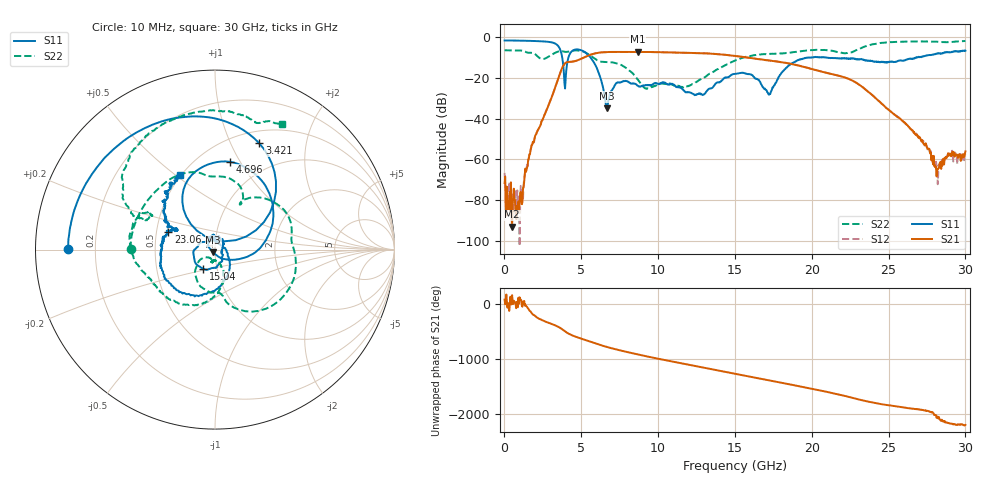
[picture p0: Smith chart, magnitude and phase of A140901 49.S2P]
!  2-Port S-parameters saved by WinCal
! VAR MeasName=S-Parameters (CALIBRATED_DATA) read from VNA (N5244A)
! VAR MeasDate=11/3/2014 9:34:34 AM
! VAR NAME=A140901 49
! VAR FILENAME=A140901 49.S2P
! VAR DATE=11/3/2014 9:34:34 AM
! VAR PHYS_PORTS=1,2
# Hz S RI R 50
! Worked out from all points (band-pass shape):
!   801 points, 10 MHz to 30 GHz, reference 50 ohm
!   highest |S21| = -7.30 dB at 8.67 GHz (marker M1); lowest = -93.0 dB at 497.3 MHz (marker M2)
!   |S21| within 3 dB of the highest: 5.111 GHz to 16 GHz (10.89 GHz wide, 103 % of centre)
!   lowest |S11| = -35.0 dB at 6.645 GHz (marker M3), VSWR 1.04, Z = 49 - j1.43 ohm
!   |S11| at or under -10 dB: 3.757 GHz to 4.167 GHz (410 MHz wide, 10.4 % of centre); 5.593 GHz to 20.06 GHz (14.47 GHz wide, 113 % of centre); 20.8 GHz to 26.84 GHz (6.04 GHz wide, 25.4 % of centre)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
!   |S22| runs from -25.4 to -2.0 dB; largest |S21 - S12| = 0.0038
!   S11 on the Smith chart (normalised r, x): 10 MHz: 0.10, +0.00; 3.421 GHz: 0.64, +1.29; 4.696 GHz: 0.70, +0.90; 15.04 GHz: 0.86, -0.19; 23.06 GHz: 0.58, +0.12; 30 GHz: 0.49, +0.52
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1e7  -0.8177 0.00209  7.3e-06 0.000264  0.00033 0.000331  -0.4708 0.00438
4.973375e8  -0.7992 0.1616  -2.19e-05 4.15e-06  -5.05e-05 0.000124  -0.4113 0.2191
1.05965e9  -0.7361 0.3355  6.56e-06 0.00016  1.52e-05 0.000224  -0.2331 0.402
1.734425e9  -0.6 0.526  -0.00154 -0.00114  -0.00151 -0.00119  0.0341 0.4071
3.421362e9  0.2467 0.5922  0.0621 -0.0466  0.0623 -0.0466  0.3434 0.2548
3.946188e9  -0.0046 0.0543  -0.1504 -0.1685  -0.1507 -0.1682  0.4259 0.0644
4.695938e9  0.0815 0.4893  -0.1515 0.2138  -0.1513 0.2136  0.4282 -0.1876
5.033325e9  0.257 0.3878  -0.0136 0.2958  -0.0139 0.2952  0.3298 -0.3053
5.933025e9  0.1966 -0.031  0.3938 0.0516  0.3934 0.0523  0.0544 -0.2786
6.645288e9  -0.0103 -0.0146  0.253 -0.3406  0.253 -0.3401  0.0115 -0.2409
8.669612e9  -0.000731 0.0642  -0.4232 0.0849  -0.4227 0.0843  -0.0753 -0.0505
1.001916e10  0.00609 0.0707  0.00649 0.4235  0.0065 0.4224  -0.0168 -0.0671
1.155615e10  0.0455 0.0284  0.4084 0.0303  0.4084 0.0308  -0.00548 -0.0591
1.305565e10  0.0363 -0.0202  0.0878 -0.3873  0.0867 -0.3867  0.0362 -0.0971
1.5005e10  -0.0603 -0.1082  -0.3412 0.0266  -0.3407 0.0278  -0.00464 -0.2635
1.504249e10  -0.0647 -0.1073  -0.3388 0.0383  -0.3387 0.0393  -0.0104 -0.265
1.725425e10  0.027 0.0301  0.1485 0.2191  0.1455 0.2185  -0.301 -0.2388
2.002832e10  -0.2529 -0.1863  -0.0279 -0.1599  -0.0272 -0.1609  -0.4734 0.0296
2.306481e10  -0.2601 0.0985  0.0264 0.0628  0.0261 0.0634  -0.4611 0.1994
2.501416e10  -0.211 0.1129  0.0128 -0.0101  0.0129 -0.0102  -0.3863 0.6314
2.812562e10  -0.2842 0.2622  -1.8e-05 0.00038  -0.000219 0.000646  0.1641 0.7458
3e10  -0.1964 0.416  0.00127 -0.000909  0.000988 -0.000972  0.3735 0.7007
